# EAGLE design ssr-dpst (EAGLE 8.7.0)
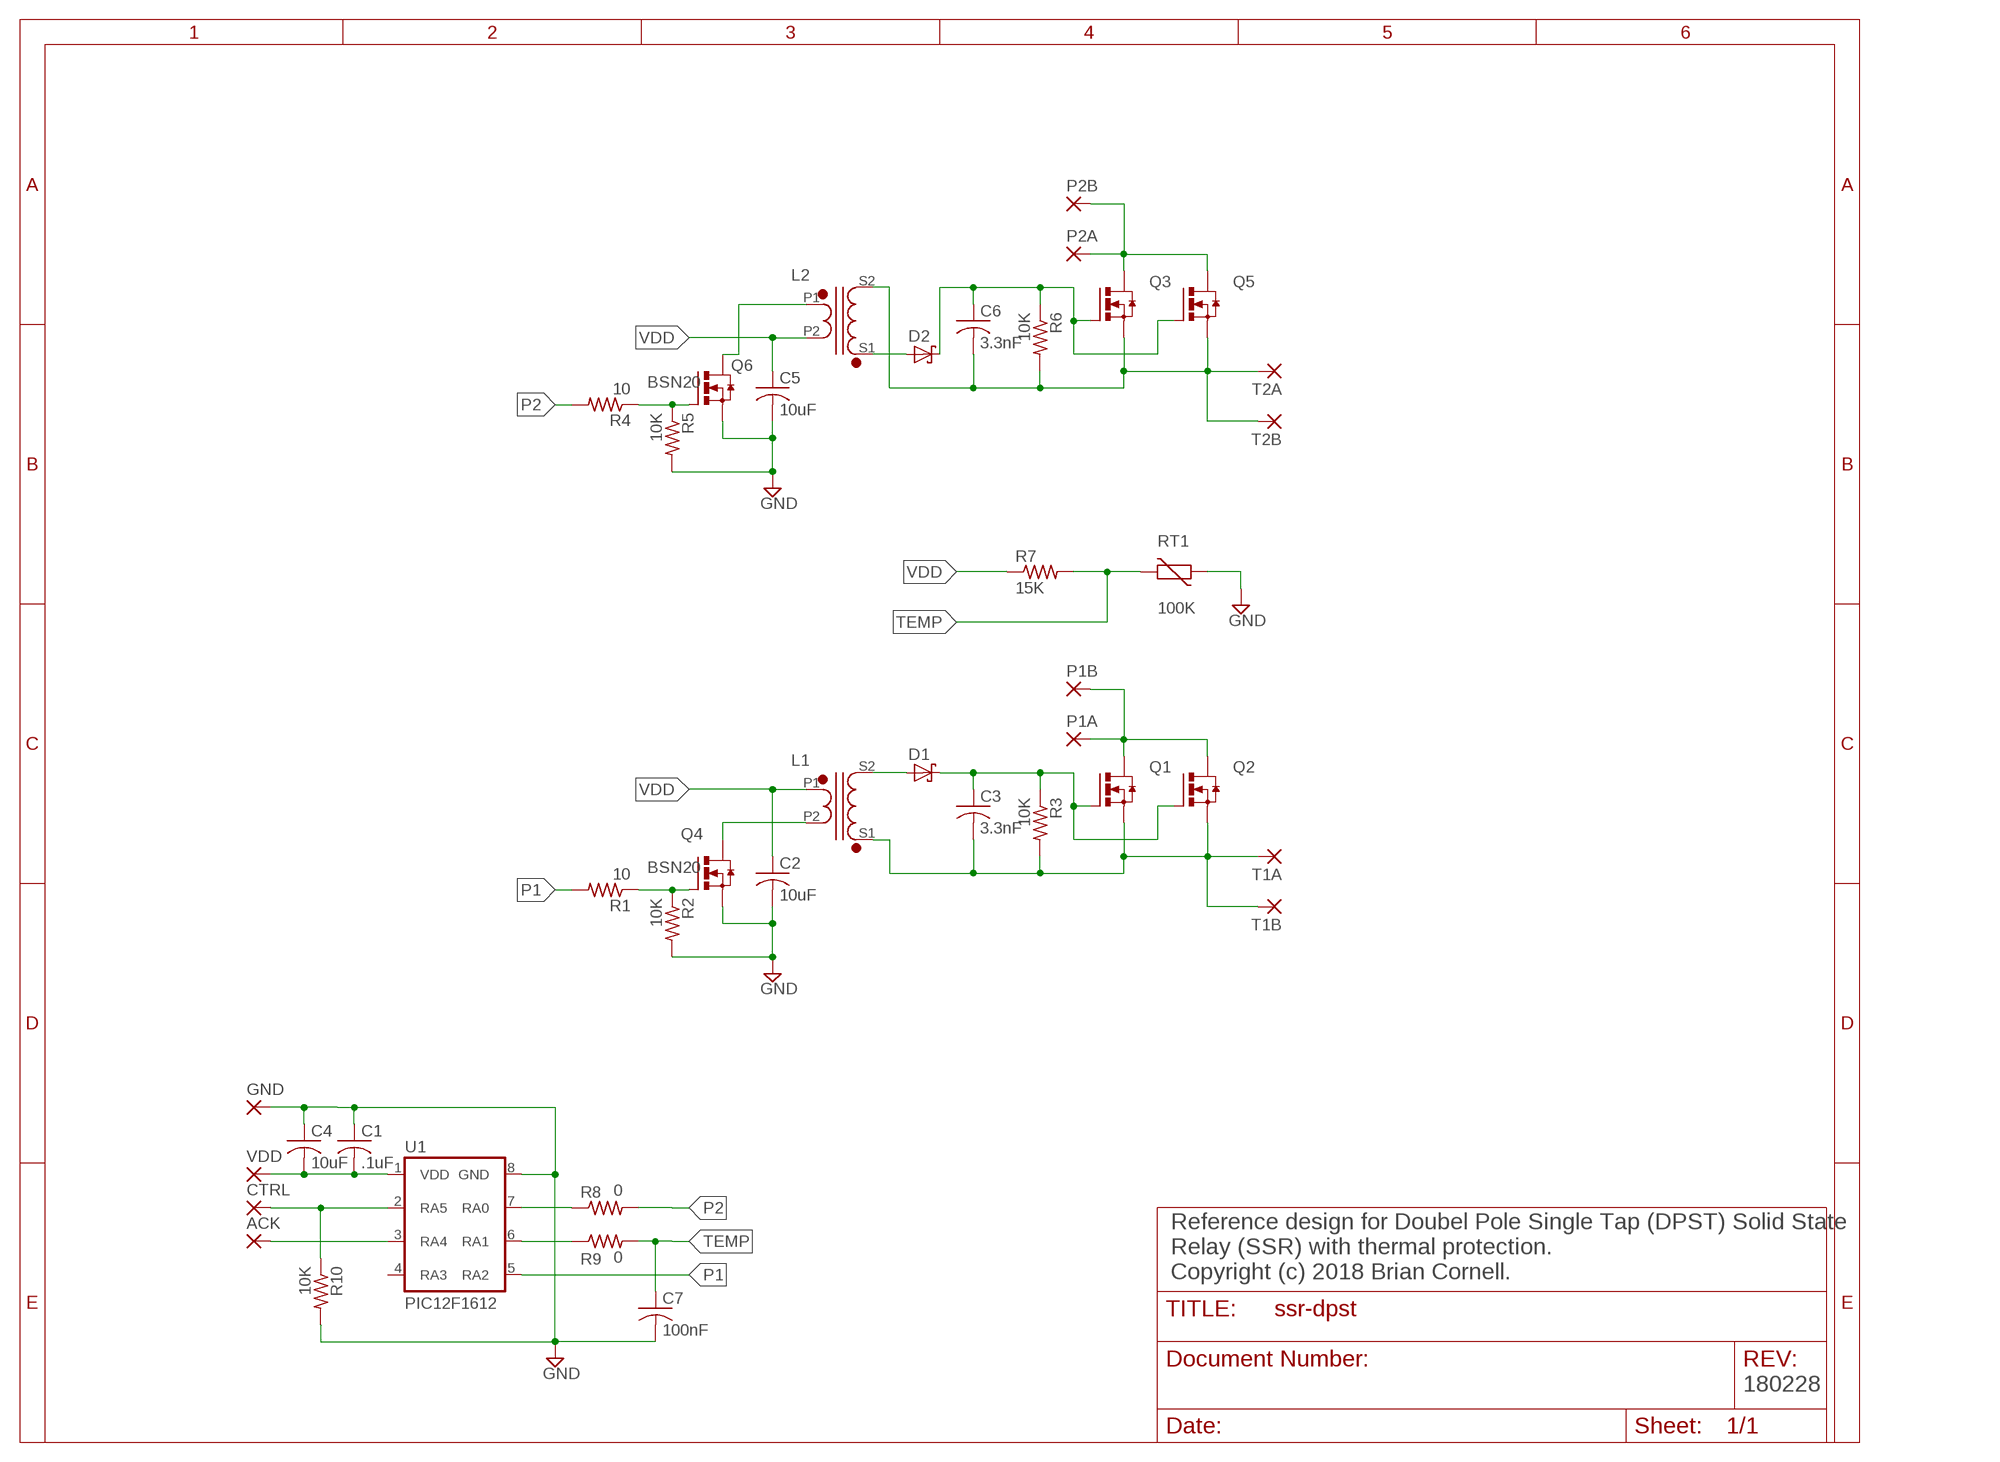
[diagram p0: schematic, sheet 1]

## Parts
ACK  PAD.65M  [PAD-RND-AUTO/.65-M]
C1  .1uF  C-USC0805  [C0805]
C2  10uF  C-USC1206  [C1206]
C3  3.3nF  C-USC0805  [C0805]
C4  10uF  C-USC1206  [C1206]
C5  10uF  C-USC1206  [C1206]
C6  3.3nF  C-USC0805  [C0805]
C7  100nF  C-USC0805  [C0805]
CTRL  PAD.65M  [PAD-RND-AUTO/.65-M]
D1  SCHOTTKYSOD123  [SOD123]
D2  SCHOTTKYSOD123  [SOD123]
GND  PAD.65M  [PAD-RND-AUTO/.65-M]
L1  FB_P1_S1HT  [TOROID-FLYBACK-B64290P0037X087-H]
L2  FB_P1_S1HT  [TOROID-FLYBACK-B64290P0037X087-H]
P1A  PAD.0635  [.15/.0635]
P1B  PAD.0635  [.15/.0635]
P2A  PAD.0635  [.15/.0635]
P2B  PAD.0635  [.15/.0635]
Q1  NFETTO263-7106  [TO-263-7106]
Q2  NFETTO263-7106  [TO-263-7106]
Q3  NFETTO263-7106  [TO-263-7106]
Q4  BSN20  [SOT23]
Q5  NFETTO263-7106  [TO-263-7106]
Q6  BSN20  [SOT23]
R1  10  R-US_R0805  [R0805]
R2  10K  R-US_R0805  [R0805]
R3  10K  R-US_R0805  [R0805]
R4  10  R-US_R0805  [R0805]
R5  10K  R-US_R0805  [R0805]
R6  10K  R-US_R0805  [R0805]
R7  15K  R-US_R0805  [R0805]
R8  0  R-US_R0805  [R0805]
R9  0  R-US_R0805  [R0805]
R10  10K  R-US_R0805  [R0805]
RT1  100K  NTC805  [R0805]
T1A  PAD.0635  [.15/.0635]
T1B  PAD.0635  [.15/.0635]
T2A  PAD.0635  [.15/.0635]
T2B  PAD.0635  [.15/.0635]
U1  PIC12F1612  PIC12F161XSO08  [SO08]
VDD  PAD.65M  [PAD-RND-AUTO/.65-M]

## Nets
CTRL: CTRL.P$1(P) R10.1 U1.2(RA5)
GATE1: C3.1 D1.C Q1.1(G) Q2.1(G) R3.1
GATE2: C6.1 D2.C Q3.1(G) Q5.1(G) R6.1
GND: C1.1 C2.2 C4.1 C5.2 C7.2 GND.P$1(P) Q4.2(S) Q6.2(S) R2.2 R5.2 R10.2 RT1.1 U1.8(GND)
N$1: L2.P1 Q6.3(D)
N$2: ACK.P$1(P) U1.3(RA4)
N$6: L1.P2 Q4.3(D)
N$7: Q6.1(G) R4.1 R5.1
N$8: Q4.1(G) R1.1 R2.1
N$9: D2.A L2.S1
N$11: D1.A L1.S2
P1: R1.2 U1.5(RA2)
P1IN: P1A.1(P) P1B.1(P) Q1.2(D) Q2.2(D)
P1OUT: C3.2 L1.S1 Q1.3(S) Q2.3(S) R3.2 T1A.1(P) T1B.1(P)
P2: R4.2 R8.2
P2IN: P2A.1(P) P2B.1(P) Q3.2(D) Q5.2(D)
P2J: R8.1 U1.7(RA0)
P2OUT: C6.2 L2.S2 Q3.3(S) Q5.3(S) R6.2 T2A.1(P) T2B.1(P)
TEMP: C7.1 R7.2 R9.2 RT1.2
TEMPJ: R9.1 U1.6(RA1)
VDD: C1.2 C2.1 C4.2 C5.1 L1.P1 L2.P2 R7.1 U1.1(VDD) VDD.P$1(P)
Unconnected: U1.4(RA3)

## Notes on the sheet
- Reference design for Doubel Pole Single Tap (DPST) Solid State
  Relay (SSR) with thermal protection.
  Copyright (c) 2018 Brian Cornell.
- 180228

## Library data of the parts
ACK CTRL GND P1A P1B P2A P2B T1A T1B T2A T2B VDD = brian:PAD
C1-C7 = rcl:C-US: CAPACITOR, American symbol; SPICEPREFIX: C
D1 D2 = brian:SCHOTTKY
L1 L2 = brian:FB_P1_S1
Q1-Q3 Q5 = brian:NFET
Q4 Q6 = brian:BSN20: Diodes Inc. N-CHANNEL ENHANCEMENT MODE FIELD MOSFET Product Summary Description This new generation MOSFET has been designed to minimize the on- state resistance (RDS(ON)) and yet maintain superior switching performance, making it ideal for high efficiency power management applications. BSN20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
R1-R10 = rcl:R-US_: RESISTOR, American symbol; SPICEPREFIX: R
RT1 = brian:NTC: NTC Thermistor
U1 = brian:PIC12F161X: PIC12F1612/13 8-bit MPU

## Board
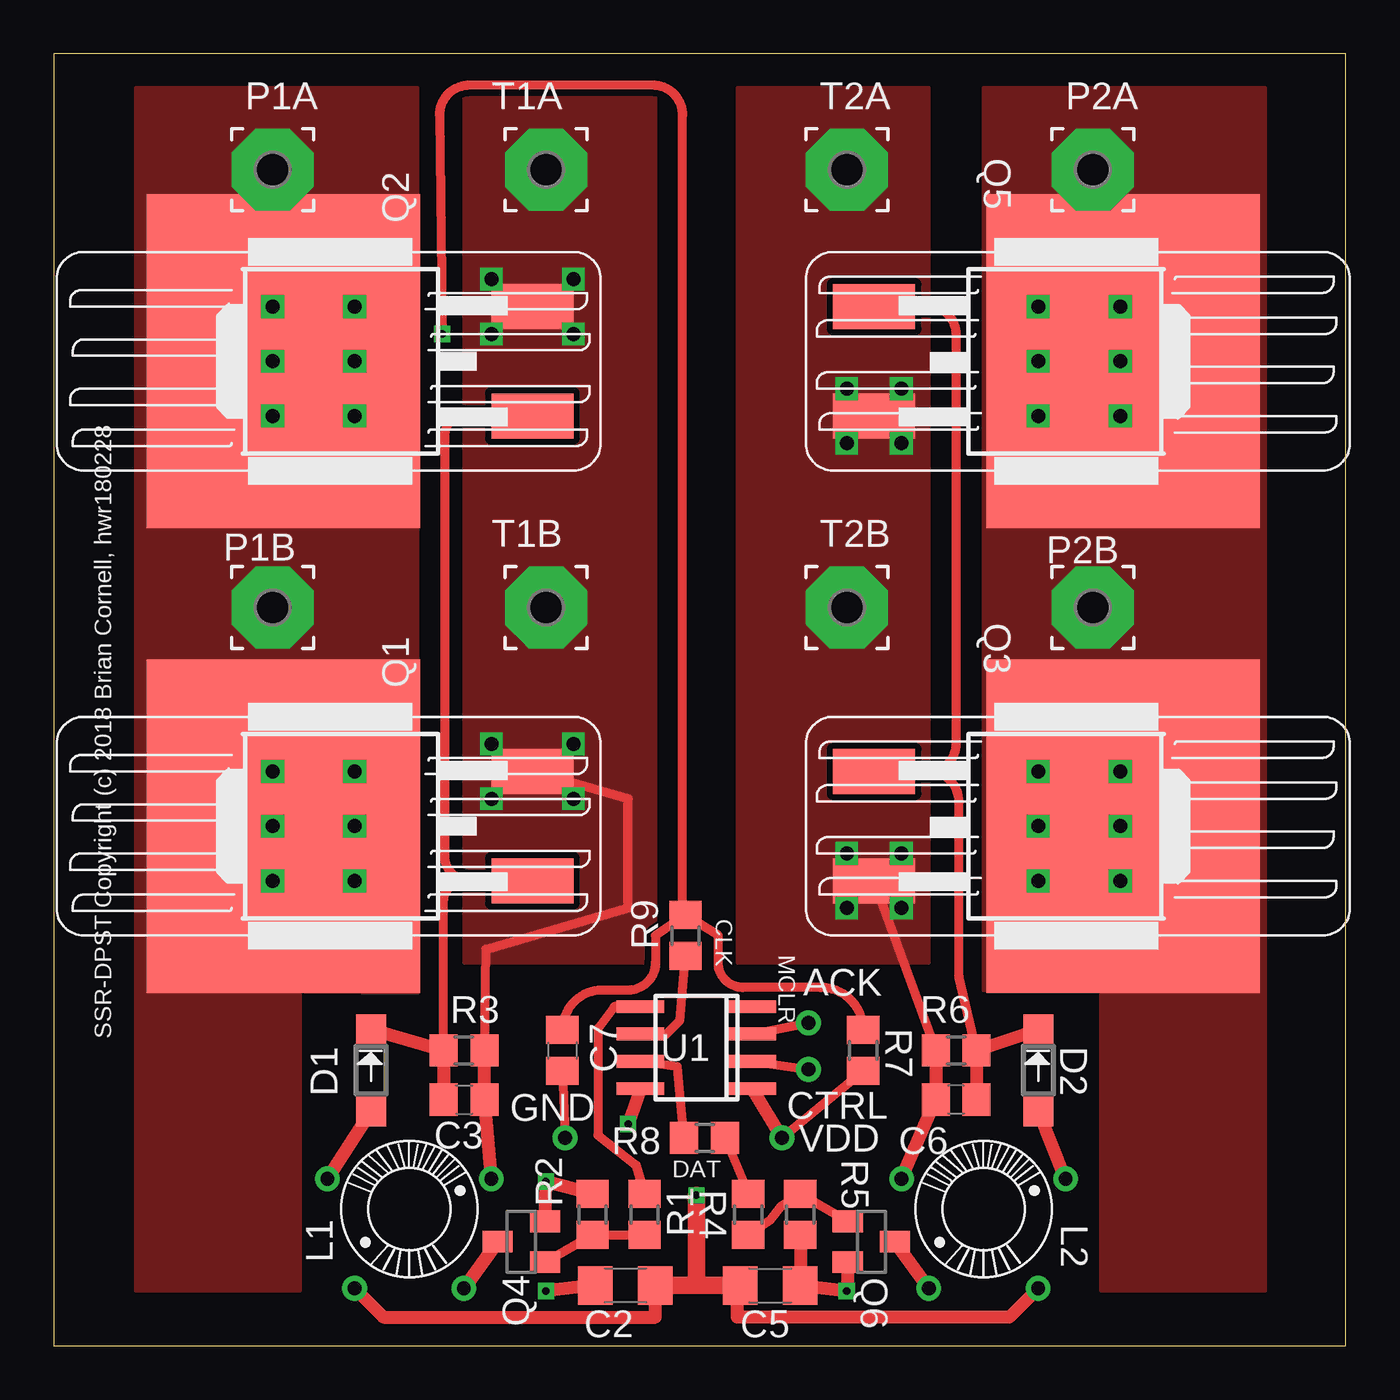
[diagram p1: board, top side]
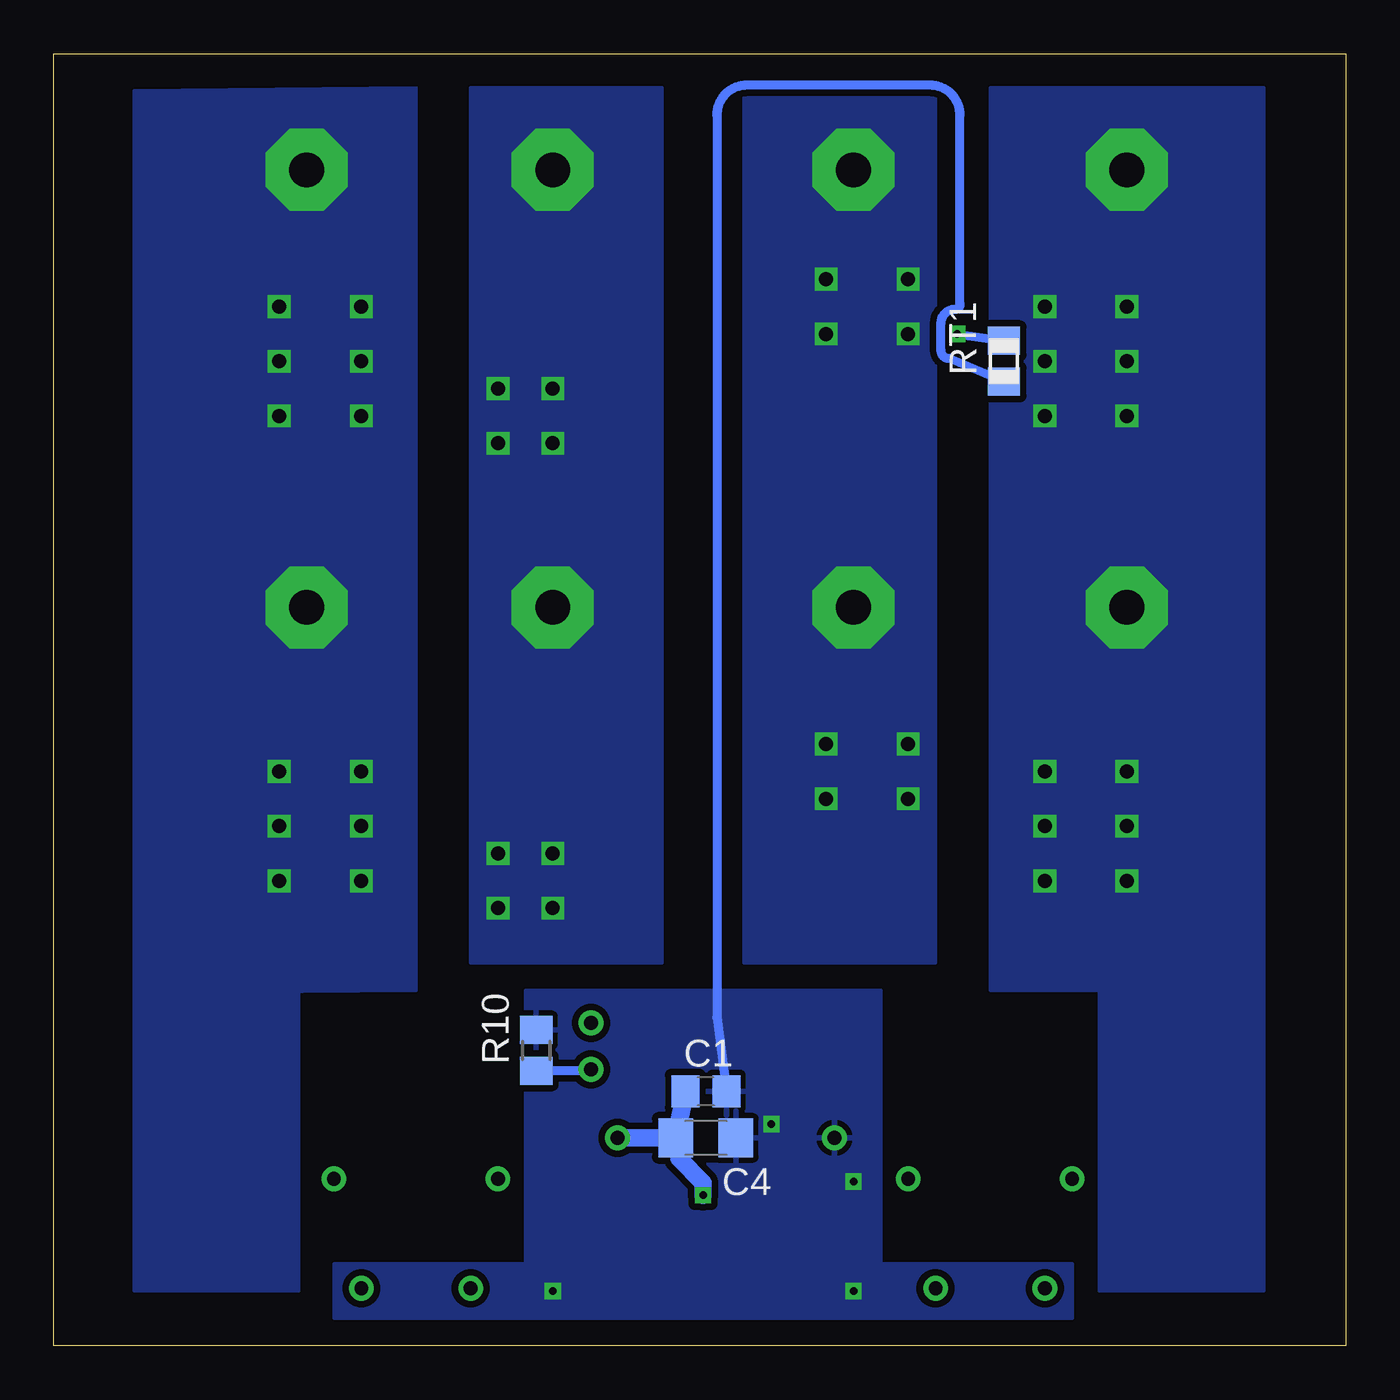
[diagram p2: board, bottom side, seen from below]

Size 60 x 60 mm. Coordinates in mm from the lower left corner, seen from the top.
Outline: 0,0 60,0 60,60 0,60 0,0
Copper layers (1*16): Top 0.035mm / dielectric 1.5mm / Bottom 0.035mm
Design rules "default": minimum track width 6mil, minimum drill 0.35mm, track to track 6mil, track to pad 6mil, pad to pad 6mil, via to via 6mil, smd to smd 6mil, copper to edge 40mil, drill to drill 6mil, minimum pad ring 10mil, minimum via ring 8mil, stop-mask expansion 4mil, vias tented up to drill 0mil, thermal gap 10mil
bRestrict: area 29.2,8.9 to 30.5,10.2

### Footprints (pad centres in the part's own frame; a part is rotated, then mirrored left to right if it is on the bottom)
PAD-RND-AUTO/.65-M = drill 0.65: P$1 0,0
C0805 = smd 1.3 x 1.5: 1 -0.95,0; 2 0.95,0
C1206 = smd 1.6 x 1.8: 1 -1.4,0; 2 1.4,0
SOD123 = smd 1.4 x 1.4: A -0.1,0; C -3.9,0
TOROID-FLYBACK-B64290P0037X087-H = drill 0.635: P1 -3.683,2.54; P2 -3.683,-2.54; S1 1.397,-3.81; S2 1.397,3.81
.15/.0635 = drill 1.613 pad 3.81 octagon: 1 0,0
TO-263-7106 = smd 2.08 x 3.81: 1 -2.54,-6.985; 3 2.54,-6.985 | smd 15.5 x 12.7: 2 0,4.572
SOT23 = smd 1 x 1.4: 1 -0.95,-1.1; 2 0.95,-1.1; 3 0,1.1
R0805 = smd 1.3 x 1.5: 1 -0.95,0; 2 0.95,0
SO08 = smd 0.6 x 2.2: 1 -1.905,-2.6; 2 -0.635,-2.6; 3 0.635,-2.6; 4 1.905,-2.6; 5 1.905,2.6; 6 0.635,2.6; 7 -0.635,2.6; 8 -1.905,2.6

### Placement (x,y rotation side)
ACK  35.05,14.99 0 top
C1  29.72,11.81 180 bottom
C2  26.54,2.79 180 top
C3  19.05,11.43 0 top
C4  29.72,9.65 180 bottom
C5  33.27,2.79 0 top
C6  41.91,11.43 180 top
C7  23.62,13.72 270 top
CTRL  35.05,12.83 0 top
D1  14.73,10.79 270 top
D2  45.72,10.79 270 top
GND  23.75,9.65 0 top
L1  16.51,6.35 90 top
L2  43.18,6.35 90 top
P1A  10.16,54.61 0 top
P1B  10.16,34.29 0 top
P2A  48.26,54.61 0 top
P2B  48.26,34.29 0 top
Q1  15.24,24.13 90 top
Q2  15.24,45.72 90 top
Q3  45.09,24.13 270 top
Q4  21.72,4.83 90 top
Q5  45.09,45.72 270 top
Q6  37.97,4.83 270 top
R1  27.43,6.1 90 top
R2  25.02,6.1 90 top
R3  19.05,13.72 0 top
R4  32.26,6.1 90 top
R5  34.67,6.1 270 top
R6  41.91,13.72 180 top
R7  37.59,13.72 90 top
R8  30.23,9.65 0 top
R9  29.34,19.05 90 top
R10  37.59,13.72 90 bottom
RT1  15.88,45.72 90 bottom
T1A  22.86,54.61 0 top
T1B  22.86,34.29 0 top
T2A  36.83,54.61 0 top
T2B  36.83,34.29 0 top
U1  29.84,13.84 90 top
VDD  33.82,9.65 0 top

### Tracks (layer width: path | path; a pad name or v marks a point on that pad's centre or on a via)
CTRL
  Top 0.406: U1.2 CTRL.P$1
  Bottom 0.406: CTRL.P$1 35.11,12.77 R10.1
GATE1
  Top 0.406: R3.1 18.1,20.64 arc-90 19.05,21.59 Q1.1 19.3,21.59 arc-90 18.16,22.73 18.16,42.29 arc-90 19.05,43.18 Q2.1
  Top 0.61: D1.C R3.1 C3.1
GATE2
  Top 0.406: R6.1 42.04,17.14 42.04,25.27 arc90 40.64,26.67 | 40.64,26.67 Q3.1 40.64,26.67 | 40.64,26.67 arc90 41.91,27.94 41.91,46.99 arc90 40.64,48.26 Q5.1
  Top 0.61: C6.1 R6.1 D2.C
GND  (via drill 0.35)
  Top 0.406: C7.2 GND.P$1
  Top 0.61: Q4.2 v22.86,7.62 R2.2 | Q6.2 v36.83,2.54 C5.2 R5.2 | C2.2 v22.86,2.54 | U1.8 v26.67,10.29
  Bottom 0.406: RT1.1 18.41,45.85 arc90 18.8,46.23 18.8,47.5 arc90 18.16,48.13 arc-90 17.91,48.39 17.91,57.15 arc-90 19.3,58.55 27.81,58.55 arc-90 29.21,57.15 29.21,15.24 C1.1
  pour Bottom (isolate 0.305): 12.7,1.27 46.99,1.27 46.99,3.81 38.1,3.81 38.1,16.51 21.59,16.51 21.59,3.81 12.7,3.81
N$1
  Top 0.61: Q6.3 L2.P1
N$2
  Top 0.406: U1.3 ACK.P$1
N$6
  Top 0.61: Q4.3 L1.P2
N$7
  Top 0.406: Q6.1 R5.1 33.78,6.48 33.27,5.84 R4.1
N$8
  Top 0.406: Q4.1 R2.1 R1.1
N$9
  Top 0.61: L2.S1 D2.A
N$11
  Top 0.61: D1.A L1.S2
P1
  Top 0.406: U1.5 26.04,15.75 25.27,14.73 25.27,9.78 27.05,8.38 R1.2
P1IN  (via drill 0.65)
  other vias: 10.16,21.59 13.97,21.59 13.97,26.67 10.16,26.67 10.16,48.26 10.16,43.18 13.97,43.18 13.97,48.26 10.16,24.13 13.97,24.13 13.97,45.72 10.16,45.72
  pour Top (isolate 0.305, no thermals): 3.81,16.51 3.81,58.42 16.89,58.42 16.89,16.38
  pour Bottom (isolate 0.305, no thermals): 3.81,16.51 3.81,58.42 16.51,58.42 16.51,16.51
  pour Top (isolate 0.305, no thermals): 3.81,17.78 3.81,2.54 11.43,2.54 11.43,17.78
  pour Bottom (isolate 0.305, no thermals): 3.81,2.54 3.81,22.86 11.43,22.86 11.43,2.54
P1OUT  (via drill 0.65)
  Top 0.406: R3.2 20.07,18.41 26.67,20.32 26.67,25.4 Q1.3
  Top 0.61: L1.S1 C3.2 R3.2
  other vias: 24.13,27.94 20.32,27.94 20.32,25.4 24.13,25.4 24.13,46.99 24.13,49.53 20.32,49.53 20.32,46.99
  pour Top (isolate 0.305, no thermals): 19.05,17.78 27.94,17.78 27.94,58.42 19.05,58.42
  pour Bottom (isolate 0.305, no thermals): 19.05,17.78 27.94,17.78 27.94,58.42 19.05,58.42
P2
  Top 0.406: R8.2 R4.2
P2IN  (via drill 0.65)
  other vias: 45.72,48.26 49.53,48.26 49.53,45.72 49.53,43.18 45.72,43.18 45.72,45.72 45.72,26.67 45.72,24.13 45.72,21.59 49.53,21.59 49.53,24.13 49.53,26.67
  pour Top (isolate 0.305, no thermals): 43.18,16.51 43.18,58.42 56.26,58.42 56.26,16.38
  pour Top (isolate 0.305, no thermals): 48.64,17.78 48.64,2.54 56.26,2.54 56.26,17.78
  pour Bottom (isolate 0.305, no thermals): 43.18,16.51 43.18,58.42 56.26,58.29 56.26,16.38
  pour Bottom (isolate 0.305, no thermals): 48.64,22.86 48.64,2.54 56.26,2.54 56.26,22.86
P2J
  Top 0.406: R8.1 28.96,12.95 U1.7
P2OUT  (via drill 0.65)
  Top 0.406: R6.2 Q3.3
  Top 0.61: R6.2 C6.2 L2.S2
  other vias: 36.83,44.45 39.37,44.45 39.37,41.91 36.83,41.91 36.83,22.86 39.37,22.86 39.37,20.32 36.83,20.32
  pour Top (isolate 0.305, no thermals): 31.75,17.78 40.64,17.78 40.64,58.42 31.75,58.42
  pour Bottom (isolate 0.305, no thermals): 31.75,17.78 40.64,17.78 40.64,58.42 31.75,58.42
TEMP  (via drill 0.35)
  Top 0.406: R7.2 arc90 35.62,16.64 32,16.64 arc-90 30.86,17.78 30.86,19.05 R9.2 | R9.2 arc-90 29.21,20.13 29.21,57.15 arc90 27.81,58.55 21.97,58.55 19.3,58.55 arc90 17.91,57.15 18.03,47.75 v18.03,46.99 | R9.2 27.94,19.05 27.94,17.78 arc-90 26.67,16.51 25.47,16.51 arc90 C7.1
  Bottom 0.406: v18.03,46.99 RT1.2
TEMPJ
  Top 0.406: U1.6 28.45,14.48 29.08,15.11 R9.1
VDD  (via drill 0.35)
  Top 0.406: VDD.P$1 R7.1
  Top 0.61: L1.P1 15.32,1.32 27.94,1.32 C2.1 | L2.P2 44.37,1.32 31.75,1.32 31.75,2.67 C5.1 | VDD.P$1 U1.1
  Top 0.813: C2.1 29.84,2.79 | 29.84,2.79 C5.1 | v29.84,6.99 29.84,2.79
  Bottom 0.813: VDD.P$1 C4.2 | v29.84,6.99 29.84,7.57 30.96,8.69 30.96,9.5 C4.2 | C4.2 C1.2

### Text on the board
tPlace: SSR-DPST Copyright (c) 2018 Brian Cornell, hwr180228 | CLK | MCLR | DAT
